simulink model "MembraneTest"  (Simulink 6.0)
settings: Solver=ode5  StartTime=0.0  StopTime=20  FixedStep=0.001  RelTol=1e-3
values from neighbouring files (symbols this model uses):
  b = S/Sm    (= 0.1)    [Constantes.m]    (also in ConstantesBck.m)
  C = 1    [Constantes.m]    (also in ConstantesBck.m)
  Fact = 10^2    (= 100)    [Constantes.m]    (also in ConstantesBck.m)
  gk = 36    [Constantes.m]    (also in ConstantesBck.m; sim_hh.m)
  gl = 0.3    [Constantes.m]    (also in ConstantesBck.m; sim_hh.m)
  gna = 120    [Constantes.m]    (also in ConstantesBck.m; sim_hh.m)
  h0 = 0.5961    [Constantes.m]    (also in ConstantesBck.m)
  m0 = 0.0529    [Constantes.m]    (also in ConstantesBck.m)
  mK = 0    [Constantes.m]    (also in ConstantesBck.m)
  mL = 0    [Constantes.m]    (also in ConstantesBck.m)
  mNa = 0    [Constantes.m]    (also in ConstantesBck.m)
  n0 = 0.3177    [Constantes.m]    (also in ConstantesBck.m)
  Sm = 3.14e-2    (= 0.0314)    [Constantes.m]    (also in ConstantesBck.m = 0.000314)
  Vk = -82    [Constantes.m]    (also in ConstantesBck.m)
  Vl = -59    [Constantes.m]    (also in ConstantesBck.m)
  Vna = 45    [Constantes.m]    (also in ConstantesBck.m)
  Vr = -70    [Constantes.m]    (also in ConstantesBck.m)

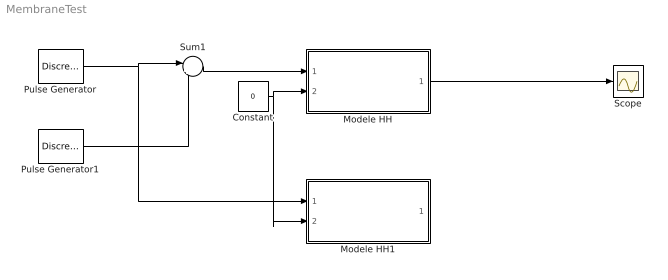
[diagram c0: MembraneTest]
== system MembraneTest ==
  Constant : Constant  Value=0
  Modele HH : Subsystem
  Modele HH1 : Subsystem
  Pulse Generator : DiscretePulseGenerator  PulseType=Time based  Amplitude=100  Period=100  PulseWidth=0.25  PhaseDelay=2
  Pulse Generator1 : DiscretePulseGenerator  PulseType=Time based  Amplitude=-100  Period=100  PulseWidth=0.25  PhaseDelay=4
  Scope : Scope
  Sum1 : Sum  Inputs=|++
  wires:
  Modele HH/1(HHout) -> Scope/1
  Constant/1 -> Modele HH/2(VRefIn), Modele HH1/2(VRefIn)
  Pulse Generator/1 -> Sum1/1, Modele HH1/1(HHin)
  Sum1/1 -> Modele HH/1(HHin)
  Pulse Generator1/1 -> Sum1/2

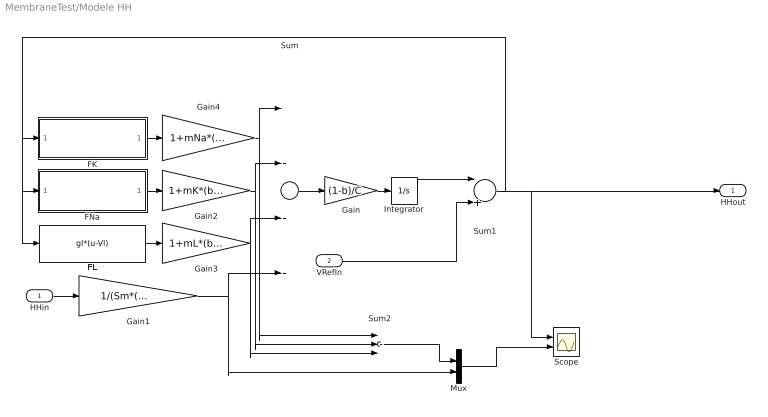
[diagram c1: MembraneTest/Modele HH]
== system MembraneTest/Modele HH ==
  HHin : Inport  Port=1  LatchInput=off
  VRefIn : Inport  Port=2  LatchInput=off
  FK : Subsystem
  FL : Fcn  Expr=gl*(u-Vl)
  FNa : Subsystem
  Gain : Gain  Gain=(1-b)/C
  Gain1 : Gain  Gain=1/(Sm*(1-b)*Fact)
  Gain2 : Gain  Gain=1+mK*(b/(1-b))
  Gain3 : Gain  Gain=1+mL*(b/(1-b))
  Gain4 : Gain  Gain=1+mNa*(b/(1-b))
  Integrator : Integrator  InitialCondition=Vr
  Mux : Mux  Inputs=2
  Scope : Scope  NumInputPorts=2
  Sum : Sum  Inputs=|---+
  Sum1 : Sum  Inputs=|++
  Sum2 : Sum  Inputs=|+++
  HHout : Outport
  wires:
  Sum/1 -> Gain/1
  Gain/1 -> Integrator/1
  FK/1(FKout) -> Gain4/1
  FNa/1(FNaOut) -> Gain2/1
  FL/1 -> Gain3/1
  HHin/1 -> Gain1/1
  Integrator/1 -> Sum1/1
  Sum1/1 -> FNa/1(FNaIn), FL/1, FK/1(FKIn), HHout/1, Scope/1
  Gain1/1 -> Sum/4, Mux/2
  Gain4/1 -> Sum/1, Sum2/1
  Gain2/1 -> Sum/2, Sum2/2
  Gain3/1 -> Sum/3, Sum2/3
  VRefIn/1 -> Sum1/2
  Sum2/1 -> Mux/1
  Mux/1 -> Scope/2

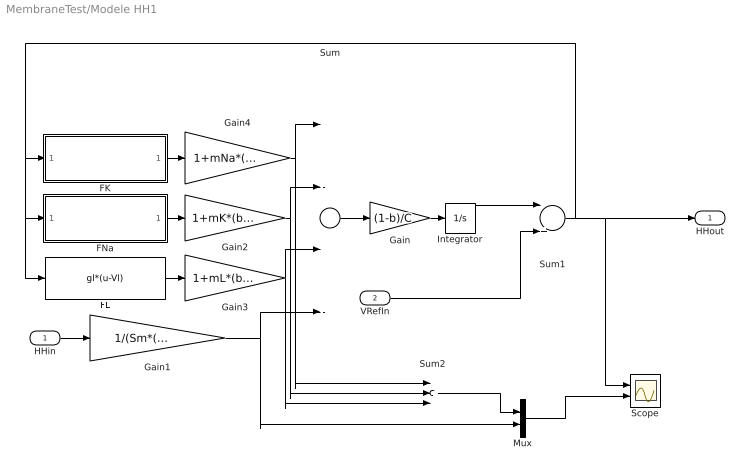
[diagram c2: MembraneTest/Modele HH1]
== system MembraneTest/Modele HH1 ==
  HHin : Inport  Port=1  LatchInput=off
  VRefIn : Inport  Port=2  LatchInput=off
  FK : Subsystem
  FL : Fcn  Expr=gl*(u-Vl)
  FNa : Subsystem
  Gain : Gain  Gain=(1-b)/C
  Gain1 : Gain  Gain=1/(Sm*(1-b)*Fact)
  Gain2 : Gain  Gain=1+mK*(b/(1-b))
  Gain3 : Gain  Gain=1+mL*(b/(1-b))
  Gain4 : Gain  Gain=1+mNa*(b/(1-b))
  Integrator : Integrator  InitialCondition=Vr
  Mux : Mux  Inputs=2
  Scope : Scope  NumInputPorts=2
  Sum : Sum  Inputs=|---+
  Sum1 : Sum  Inputs=|++
  Sum2 : Sum  Inputs=|+++
  HHout : Outport
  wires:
  Sum/1 -> Gain/1
  Gain/1 -> Integrator/1
  FK/1(FKout) -> Gain4/1
  FNa/1(FNaOut) -> Gain2/1
  FL/1 -> Gain3/1
  HHin/1 -> Gain1/1
  Integrator/1 -> Sum1/1
  Sum1/1 -> FNa/1(FNaIn), FL/1, FK/1(FKIn), HHout/1, Scope/1
  Gain1/1 -> Sum/4, Mux/2
  Gain4/1 -> Sum/1, Sum2/1
  Gain2/1 -> Sum/2, Sum2/2
  Gain3/1 -> Sum/3, Sum2/3
  VRefIn/1 -> Sum1/2
  Sum2/1 -> Mux/1
  Mux/1 -> Scope/2

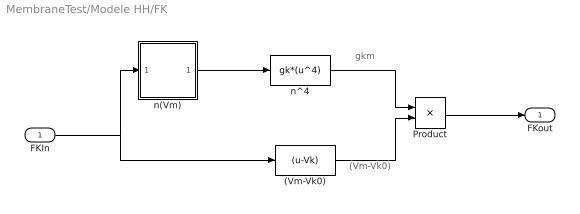
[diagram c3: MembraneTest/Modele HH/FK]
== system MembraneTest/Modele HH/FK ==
  note: gkm
  note: (Vm-Vk0)
  FKIn : Inport  Port=1  LatchInput=off
  (Vm-Vk0) : Fcn  Expr=(u-Vk)
  Product : Product
  n(Vm) : Subsystem
  n^4 : Fcn  Expr=gk*(u^4)
  FKout : Outport  InitialOutput=0
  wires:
  n(Vm)/1(n) -> n^4/1
  (Vm-Vk0)/1 -> Product/2
  Product/1 -> FKout/1
  n^4/1 -> Product/1
  FKIn/1 -> n(Vm)/1(Vm), (Vm-Vk0)/1

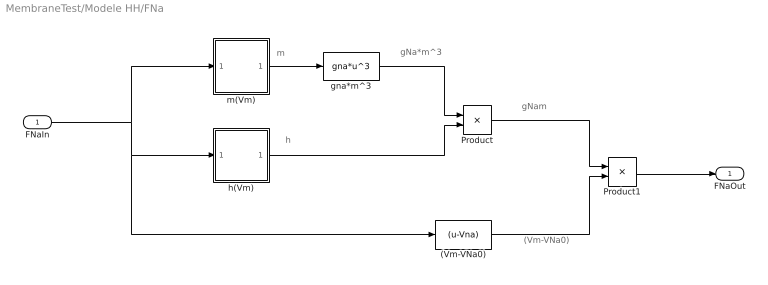
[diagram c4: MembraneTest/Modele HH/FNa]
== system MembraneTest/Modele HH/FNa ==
  note: gNa*m^3
  note: m
  note: h
  note: gNam
  note: (Vm-VNa0)
  FNaIn : Inport  Port=1  LatchInput=off
  (Vm-VNa0) : Fcn  Expr=(u-Vna)
  Product : Product
  Product1 : Product
  gna*m^3 : Fcn  Expr=gna*u^3
  h(Vm) : Subsystem
  m(Vm) : Subsystem
  FNaOut : Outport  InitialOutput=0
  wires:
  (Vm-VNa0)/1 -> Product1/2
  gna*m^3/1 -> Product/1
  Product1/1 -> FNaOut/1
  FNaIn/1 -> m(Vm)/1(Vm), h(Vm)/1(Vm), (Vm-VNa0)/1
  m(Vm)/1(n) -> gna*m^3/1
  h(Vm)/1(h) -> Product/2
  Product/1 -> Product1/1

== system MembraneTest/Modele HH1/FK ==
  note: gkm
  note: (Vm-Vk0)
  FKIn : Inport  Port=1  LatchInput=off
  (Vm-Vk0) : Fcn  Expr=(u-Vk)
  Product : Product
  n(Vm) : Subsystem
  n^4 : Fcn  Expr=gk*(u^4)
  FKout : Outport  InitialOutput=0
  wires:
  n(Vm)/1(n) -> n^4/1
  (Vm-Vk0)/1 -> Product/2
  Product/1 -> FKout/1
  n^4/1 -> Product/1
  FKIn/1 -> n(Vm)/1(Vm), (Vm-Vk0)/1

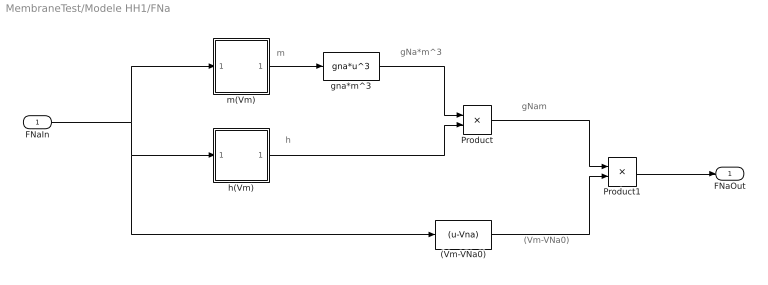
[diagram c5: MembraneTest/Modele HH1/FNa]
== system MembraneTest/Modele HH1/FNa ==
  note: gNa*m^3
  note: m
  note: h
  note: gNam
  note: (Vm-VNa0)
  FNaIn : Inport  Port=1  LatchInput=off
  (Vm-VNa0) : Fcn  Expr=(u-Vna)
  Product : Product
  Product1 : Product
  gna*m^3 : Fcn  Expr=gna*u^3
  h(Vm) : Subsystem
  m(Vm) : Subsystem
  FNaOut : Outport  InitialOutput=0
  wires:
  (Vm-VNa0)/1 -> Product1/2
  gna*m^3/1 -> Product/1
  Product1/1 -> FNaOut/1
  FNaIn/1 -> m(Vm)/1(Vm), h(Vm)/1(Vm), (Vm-VNa0)/1
  m(Vm)/1(n) -> gna*m^3/1
  h(Vm)/1(h) -> Product/2
  Product/1 -> Product1/1

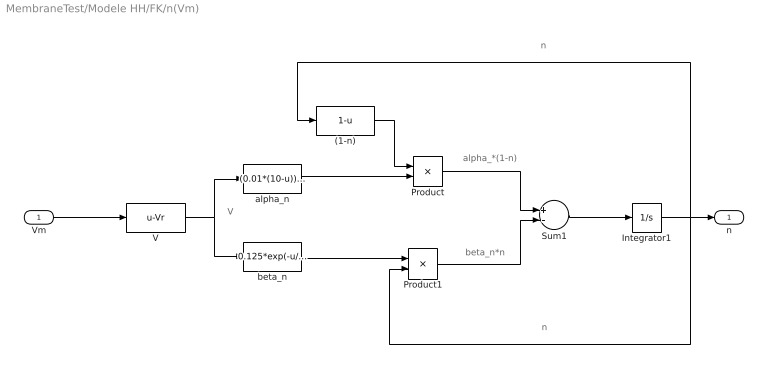
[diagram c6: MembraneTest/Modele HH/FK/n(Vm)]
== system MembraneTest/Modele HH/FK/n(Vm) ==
  note: V
  note: alpha_*(1-n)
  note: beta_n*n
  note: n
  note: n
  Vm : Inport  Port=1  LatchInput=off
  (1-n) : Fcn  Expr=1-u
  Integrator1 : Integrator  InitialCondition=n0
  Product : Product
  Product1 : Product
  Sum1 : Sum  Inputs=+-
  V : Fcn  Expr=u-Vr
  alpha_n : Fcn  Expr=(0.01*(10-u))/(exp((10-u)/10)-1)
  beta_n : Fcn  Expr=0.125*exp(-u/80)
  n : Outport  InitialOutput=0
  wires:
  V/1 -> alpha_n/1, beta_n/1
  alpha_n/1 -> Product/2
  (1-n)/1 -> Product/1
  beta_n/1 -> Product1/1
  Product/1 -> Sum1/1
  Product1/1 -> Sum1/2
  Sum1/1 -> Integrator1/1
  Integrator1/1 -> (1-n)/1, Product1/2, n/1
  Vm/1 -> V/1

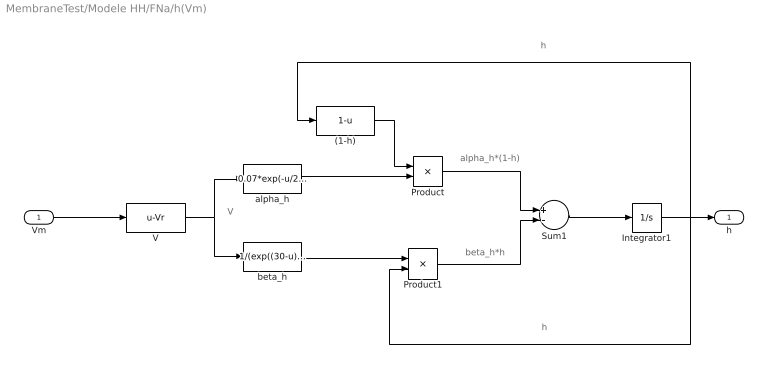
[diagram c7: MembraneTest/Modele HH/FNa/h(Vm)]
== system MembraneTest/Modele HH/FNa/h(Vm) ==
  note: h
  note: h
  note: beta_h*h
  note: alpha_h*(1-h)
  note: V
  Vm : Inport  Port=1  LatchInput=off
  (1-h) : Fcn  Expr=1-u
  Integrator1 : Integrator  InitialCondition=h0
  Product : Product
  Product1 : Product
  Sum1 : Sum  Inputs=+-
  V : Fcn  Expr=u-Vr
  alpha_h : Fcn  Expr=0.07*exp(-u/20)
  beta_h : Fcn  Expr=1/(exp((30-u)/10)+1)
  h : Outport  InitialOutput=0
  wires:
  Vm/1 -> V/1
  Integrator1/1 -> h/1, Product1/2, (1-h)/1
  Sum1/1 -> Integrator1/1
  Product1/1 -> Sum1/2
  Product/1 -> Sum1/1
  beta_h/1 -> Product1/1
  (1-h)/1 -> Product/1
  alpha_h/1 -> Product/2
  V/1 -> beta_h/1, alpha_h/1

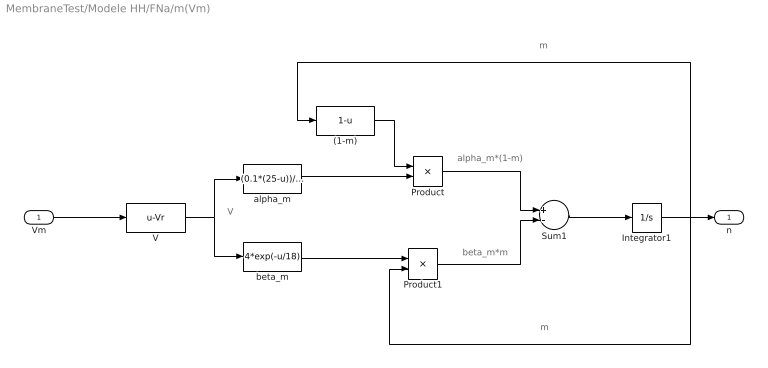
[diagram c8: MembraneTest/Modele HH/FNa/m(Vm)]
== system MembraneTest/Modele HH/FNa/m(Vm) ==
  note: m
  note: m
  note: beta_m*m
  note: alpha_m*(1-m)
  note: V
  Vm : Inport  Port=1  LatchInput=off
  (1-m) : Fcn  Expr=1-u
  Integrator1 : Integrator  InitialCondition=m0
  Product : Product
  Product1 : Product
  Sum1 : Sum  Inputs=+-
  V : Fcn  Expr=u-Vr
  alpha_m : Fcn  Expr=(0.1*(25-u))/(exp((25-u)/10)-1)
  beta_m : Fcn  Expr=4*exp(-u/18)
  n : Outport  InitialOutput=0
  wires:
  Vm/1 -> V/1
  Integrator1/1 -> n/1, Product1/2, (1-m)/1
  Sum1/1 -> Integrator1/1
  Product1/1 -> Sum1/2
  Product/1 -> Sum1/1
  beta_m/1 -> Product1/1
  (1-m)/1 -> Product/1
  alpha_m/1 -> Product/2
  V/1 -> beta_m/1, alpha_m/1

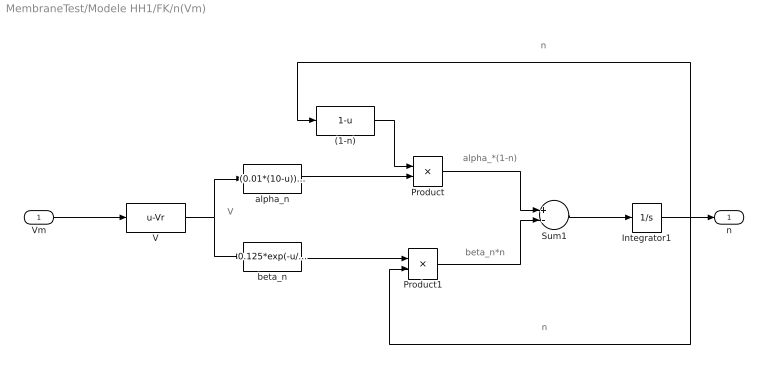
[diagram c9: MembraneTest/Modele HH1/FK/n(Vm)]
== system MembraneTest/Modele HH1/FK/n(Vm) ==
  note: V
  note: alpha_*(1-n)
  note: beta_n*n
  note: n
  note: n
  Vm : Inport  Port=1  LatchInput=off
  (1-n) : Fcn  Expr=1-u
  Integrator1 : Integrator  InitialCondition=n0
  Product : Product
  Product1 : Product
  Sum1 : Sum  Inputs=+-
  V : Fcn  Expr=u-Vr
  alpha_n : Fcn  Expr=(0.01*(10-u))/(exp((10-u)/10)-1)
  beta_n : Fcn  Expr=0.125*exp(-u/80)
  n : Outport  InitialOutput=0
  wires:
  V/1 -> alpha_n/1, beta_n/1
  alpha_n/1 -> Product/2
  (1-n)/1 -> Product/1
  beta_n/1 -> Product1/1
  Product/1 -> Sum1/1
  Product1/1 -> Sum1/2
  Sum1/1 -> Integrator1/1
  Integrator1/1 -> (1-n)/1, Product1/2, n/1
  Vm/1 -> V/1

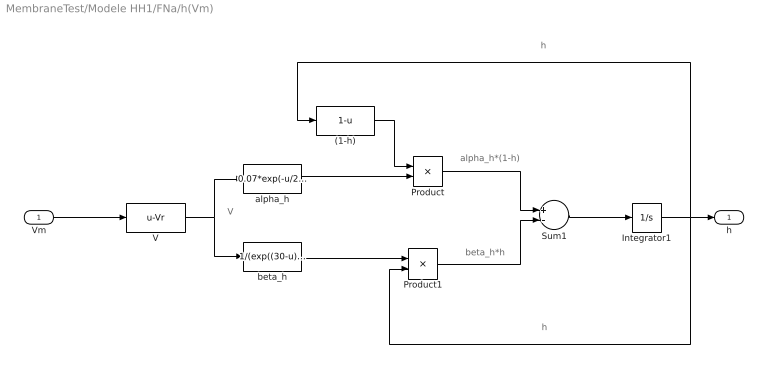
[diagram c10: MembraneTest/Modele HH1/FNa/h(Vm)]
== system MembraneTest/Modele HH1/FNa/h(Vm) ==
  note: h
  note: h
  note: beta_h*h
  note: alpha_h*(1-h)
  note: V
  Vm : Inport  Port=1  LatchInput=off
  (1-h) : Fcn  Expr=1-u
  Integrator1 : Integrator  InitialCondition=h0
  Product : Product
  Product1 : Product
  Sum1 : Sum  Inputs=+-
  V : Fcn  Expr=u-Vr
  alpha_h : Fcn  Expr=0.07*exp(-u/20)
  beta_h : Fcn  Expr=1/(exp((30-u)/10)+1)
  h : Outport  InitialOutput=0
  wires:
  Vm/1 -> V/1
  Integrator1/1 -> h/1, Product1/2, (1-h)/1
  Sum1/1 -> Integrator1/1
  Product1/1 -> Sum1/2
  Product/1 -> Sum1/1
  beta_h/1 -> Product1/1
  (1-h)/1 -> Product/1
  alpha_h/1 -> Product/2
  V/1 -> beta_h/1, alpha_h/1

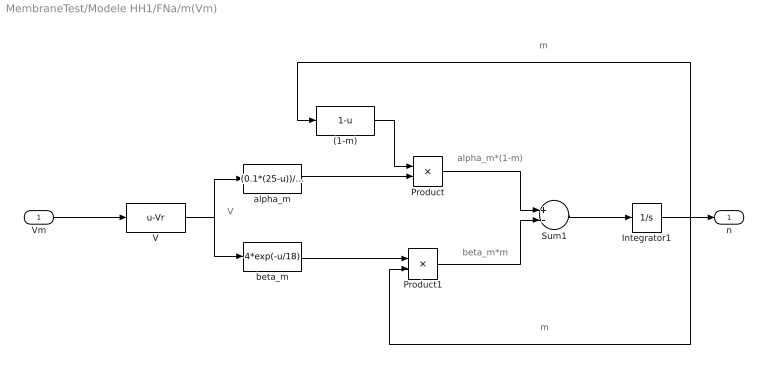
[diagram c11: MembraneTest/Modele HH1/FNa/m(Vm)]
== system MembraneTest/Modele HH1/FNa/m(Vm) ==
  note: m
  note: m
  note: beta_m*m
  note: alpha_m*(1-m)
  note: V
  Vm : Inport  Port=1  LatchInput=off
  (1-m) : Fcn  Expr=1-u
  Integrator1 : Integrator  InitialCondition=m0
  Product : Product
  Product1 : Product
  Sum1 : Sum  Inputs=+-
  V : Fcn  Expr=u-Vr
  alpha_m : Fcn  Expr=(0.1*(25-u))/(exp((25-u)/10)-1)
  beta_m : Fcn  Expr=4*exp(-u/18)
  n : Outport  InitialOutput=0
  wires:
  Vm/1 -> V/1
  Integrator1/1 -> n/1, Product1/2, (1-m)/1
  Sum1/1 -> Integrator1/1
  Product1/1 -> Sum1/2
  Product/1 -> Sum1/1
  beta_m/1 -> Product1/1
  (1-m)/1 -> Product/1
  alpha_m/1 -> Product/2
  V/1 -> beta_m/1, alpha_m/1
